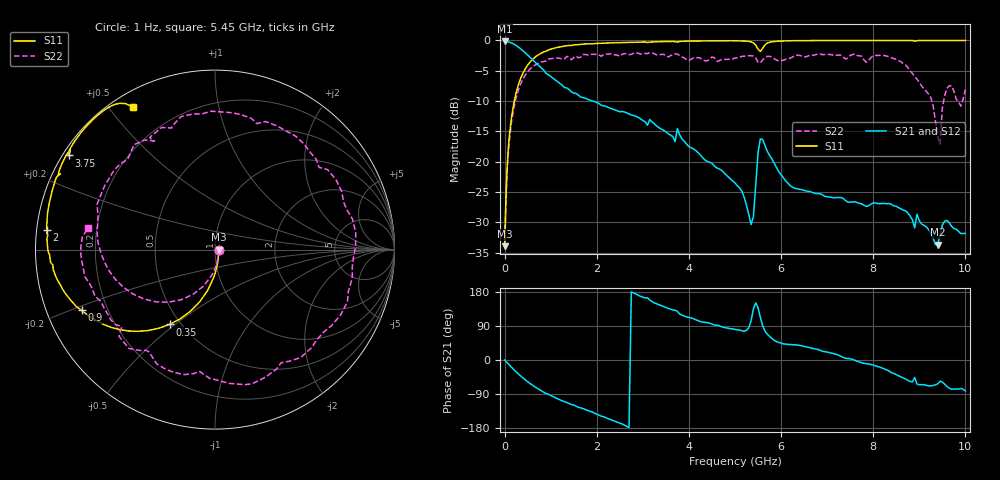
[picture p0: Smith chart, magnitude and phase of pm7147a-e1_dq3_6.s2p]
# GHz S DB R 50
! S-Parameters data
! Freq  dbS11  angS11  dbS21  angS21  dbS12  angS12  dbS22  angS22
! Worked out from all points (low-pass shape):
!   279 points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, 1 Hz to 10 GHz, reference 50 ohm
!   highest |S21| = -0.18 dB at 25.12 kHz (marker M1); lowest = -33.7 dB at 9.4 GHz (marker M2)
!   |S21| within 3 dB of the highest: start of sweep to 605 MHz
!   lowest |S11| = -34.0 dB at 25.12 kHz (marker M3), VSWR 1.04, Z = 52 - j0.00413 ohm
!   |S11| at or under -10 dB: start of sweep to 210.2 MHz
!   |S22| runs from -34.0 to -2.0 dB; largest |S21 - S12| = 5.5e-13
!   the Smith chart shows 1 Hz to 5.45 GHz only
!   S11 on the Smith chart (normalised r, x): 1 Hz: 1.04, -0.00; 350 MHz: 0.44, -0.48; 900 MHz: 0.11, -0.21; 2 GHz: 0.03, +0.06; 3.75 GHz: 0.02, +0.29; 5.45 GHz: 0.06, +0.58
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1e-09  -33.95 -0.0  -0.18 -0.0  -0.18 -0.0  -33.95 -0.0
2.51189e-05  -33.95 -0.1  -0.18 -0.0  -0.18 -0.0  -33.95 -0.1
0.1  -16.02 -93.0  -0.29 -12.9  -0.29 -12.9  -16.76 -97.4
0.35  -6.23 -121.3  -1.40 -42.4  -1.40 -42.4  -7.15 -138.4
0.9  -1.76 -155.5  -5.44 -88.6  -5.44 -88.6  -3.38 164.2
1.7  -0.61 179.5  -9.42 -128.0  -9.42 -128.0  -2.33 104.3
2  -0.50 173.3  -10.25 -143.1  -10.25 -143.1  -2.33 78.5
2.85  -0.30 158.7  -12.53 174.0  -12.53 174.0  -2.05 6.8
3.35  -0.21 151.5  -14.39 145.8  -14.39 145.8  -2.41 -41.3
3.75  -0.27 147.2  -14.56 128.5  -14.56 128.5  -2.26 -77.5
4.55  -0.06 135.6  -20.71 92.4  -20.71 92.4  -2.85 -137.9
5.05  -0.06 128.8  -23.97 79.8  -23.97 79.8  -2.87 -162.8
5.35  -0.25 123.0  -30.38 103.8  -30.38 103.8  -2.53 178.5
5.45  -0.76 120.0  -23.84 150.8  -23.84 150.8  -2.88 170.4
5.55  -1.82 125.7  -16.24 112.7  -16.24 112.7  -3.72 171.1
6.7  -0.03 115.0  -25.15 30.2  -25.15 30.2  -2.44 122.8
7.6  -0.02 107.0  -26.62 -0.8  -26.62 -0.8  -2.23 75.3
8.35  -0.01 101.1  -26.91 -29.6  -26.91 -29.6  -2.68 22.9
8.9  -0.12 96.1  -30.92 -46.1  -30.92 -46.1  -5.96 -43.2
9.4  -0.01 93.7  -33.70 -62.8  -33.70 -62.8  -15.84 -118.4
9.55  -0.01 92.7  -29.82 -63.5  -29.82 -63.5  -9.11 -62.1
10  -0.01 89.9  -31.81 -82.1  -31.81 -82.1  -8.08 -128.2
